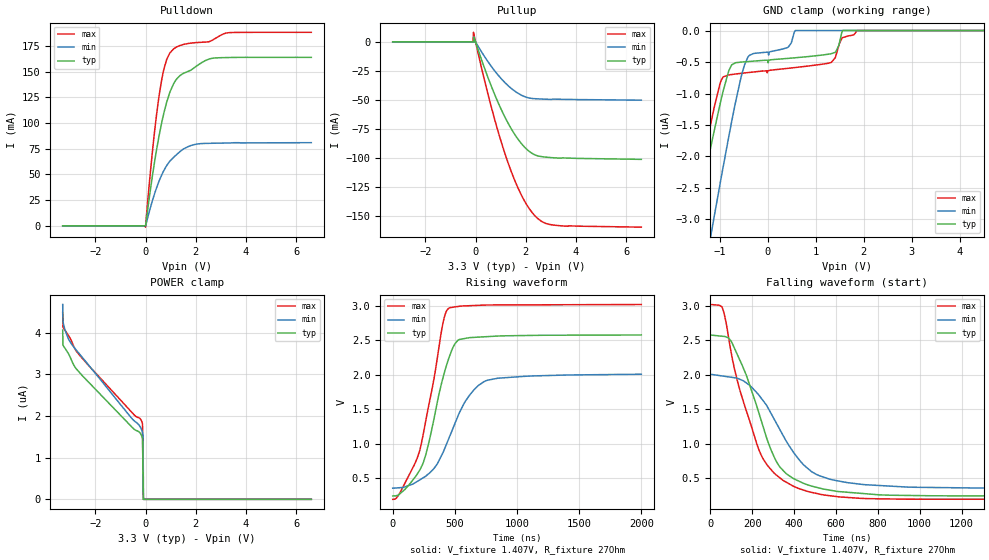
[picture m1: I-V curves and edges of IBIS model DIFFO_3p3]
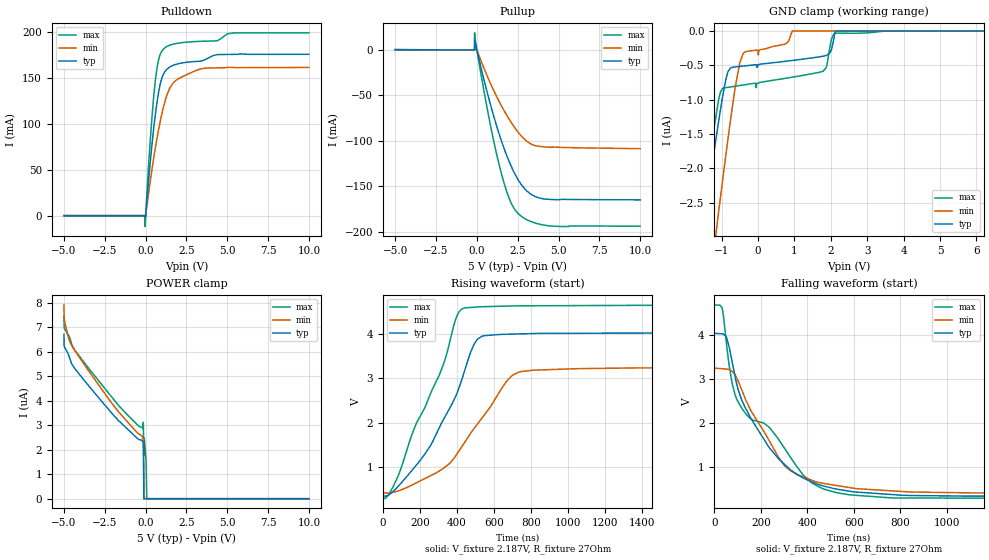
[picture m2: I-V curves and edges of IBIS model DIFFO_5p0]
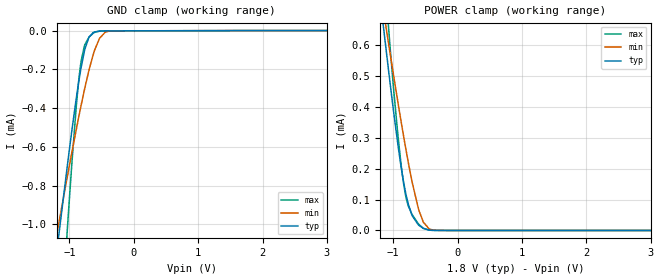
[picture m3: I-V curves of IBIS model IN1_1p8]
|Texas Instruments Incorporated
|ISO1410 5-kVRMS Isolated RS-485/RS-422 Transceiver With Robust EMC
[IBIS Ver]   4.1
[File name]   iso1410.ibs
[Date]   11/07/2018
[File Rev]   1.0
[Source]
| Texas Instruments Incorporated.
| Analog-eLab Design Center, HPA
| 12500 TI Blvd
| Dallas, TX -75243
[Notes]   Revision History:
| Rev 1.0: 11/07/2018
| - Initial version of the model
| - Model generated from simulations in SPECTRE
| - Model names with a trailing _1p8 contain the model for 1.8V operation.
|   Model names with a trailing _2p5 contain the model for 2.5V operation.
|   Model names with a trailing _3p3 contain the model for 3.3V operation.
|   Model names with a trailing _5p0 contain the model for 5.0V operation.
| - C_comp although listed in numerical order of value are
|   obtained from varying PVT conditions. For PVT conditions for
|   each specific value refer the buffer description under
|   respective [Model]. IBIS model user is responsible for using
|   appropriate C_comp to simulate for Signal Integrity.
| - For better transient results, connect a larger capactive load(100n) or
|   connect output common mode node to a constant VCM voltage.
|   typ   min   max
|   PVT 3p3   3.3   3.0   3.6
|   VCM   1.407   1.18047   1.60366
|   PVT 5p0   5.0   4.5   5.5
|   VCM   2.187   1.8289   2.4817
[Disclaimer]
| This model is designed as an aid for customers of Texas Instruments.
| TI and its licensors and suppliers make no warranties, either expressed
| or implied, with respect to this  model, including the warranties of
| merchantability or fitness for a particular purpose. The model is
| provided solely on an "as is" basis. The entire risk as to its quality
| and performance is with the customer.
| This model is subject to change without notice. Texas Instruments
| Incorporated is not responsible for updating this model.
[Copyright]
(C) Copyright 2018 Texas Instruments Incorporated.All rights reserved.
|  Component ISO1410DW 16-Pin SOIC -DW package
|  Part # ISO1410DW
[Component]   ISO1410DW
[Manufacturer]   TI
[Package]   |16 SOIC -DW package
|   typ   min   max
R_pkg   0.05   0.04   0.06
L_pkg   1.0nH   0.8nH   1.2nH
C_pkg   0.2pF   0.16pF   0.24pF
[Pin] signal_name  model_name   R_pin   L_pin   C_pin
1   VCC1   POWER   NA   NA   NA
2   GND1   GND   NA   NA   NA
3   R   OUT   NA   NA   NA
4   REB   IN1   NA   NA   NA
5   DE   IN2   NA   NA   NA
6   D   IN1   NA   NA   NA
7   NC   NC   NA   NA   NA
8   GND1   GND   NA   NA   NA
9   GND2   GND   NA   NA   NA
10   NC   NC   NA   NA   NA
11   NC   NC   NA   NA   NA
12   A   DIFFO   NA   NA   NA
13   B   DIFFO   NA   NA   NA
14   NC   NC   NA   NA   NA
15   GND2   GND   NA   NA   NA
16   VCC2   POWER   NA   NA   NA
[Diff Pin]  inv_pin  vdiff  tdelay_typ tdelay_min tdelay_max
12   13   NA   NA   NA   NA
|  Component ISO1410BDW 16-Pin SOIC -DW package
|  Part # ISO1410BDW
[Component]   ISO1410BDW
[Manufacturer]   TI
[Package]   |16 SOIC -DW package
|   typ   min   max
R_pkg   0.05   0.04   0.06
L_pkg   1.0nH   0.8nH   1.2nH
C_pkg   0.2pF   0.16pF   0.24pF
[Pin] signal_name  model_name   R_pin   L_pin   C_pin
1   VCC1   POWER   NA   NA   NA
2   GND1   GND   NA   NA   NA
3   R   OUT   NA   NA   NA
4   REB   IN1   NA   NA   NA
5   DE   IN2   NA   NA   NA
6   D   IN1   NA   NA   NA
7   NC   NC   NA   NA   NA
8   GND1   GND   NA   NA   NA
9   GND2   GND   NA   NA   NA
10   NC   NC   NA   NA   NA
11   NC   NC   NA   NA   NA
12   A   DIFFO   NA   NA   NA
13   B   DIFFO   NA   NA   NA
14   NC   NC   NA   NA   NA
15   GND2   GND   NA   NA   NA
16   VCC2   POWER   NA   NA   NA
[Diff Pin]  inv_pin  vdiff  tdelay_typ tdelay_min tdelay_max
12   13   NA   NA   NA   NA
|   Model Selectors
[Model Selector] IN1
IN1_1p8   1.8V   digital Input
IN1_2p5   2.5V   digital Input
IN1_3p3   3.3V   digital Input
IN1_5p0   5.0V   digital Input
[Model Selector] IN2
IN2_1p8   1.8V   digital Input
IN2_2p5   2.5V   digital Input
IN2_3p3   3.3V   digital Input
IN2_5p0   5.0V   digital Input
[Model Selector] OUT
OUT_1p8   1.8V   digital Output
OUT_2p5   2.5V   digital Output
OUT_3p3   3.3V   digital Output
OUT_5p0   5.0V   digital Output
[Model Selector] DIFFO
DIFFO_3p3   3.3V   Differential digital Output
DIFFO_5p0   5.0V   Differential digital Output
| Models and submodels in the file (14): DIFFO_3p3 (3-state), DIFFO_5p0 (3-state), IN1_1p8 (Input), IN1_2p5 (Input), IN1_3p3 (Input), IN1_5p0 (Input), IN2_1p8 (Input), IN2_2p5 (Input), IN2_3p3 (Input), IN2_5p0 (Input), OUT_1p8 (3-state), OUT_2p5 (3-state), OUT_3p3 (3-state), OUT_5p0 (3-state)
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|   DIFFO_3p3 Model
[Model]   DIFFO_3p3
Model_type   3-state
Polarity   Non-Inverting
Vmeas = 1.407
Vref = 1.407
Cref = 2pF
Rref = 27
|   typ   min   max
C_comp   26.160pF   24.414pF   26.499pF
|  Where Nom  PVT is Nominal Process, 3.3V,   27C
|   Fast PVT is Strong Process,  3.6,   -40C
|   Slow PVT is Weak Process,   3.0V,   150C
[Voltage Range]   3.3   3   3.6
|Junction temperature
[Temperature Range]   27   150   -40
[Pullup Reference]   3.3   3   3.6
[Pulldown Reference]   0   0   -0
[Power Clamp Reference]   3.3   3   3.6
[GND Clamp Reference]   0   0   0
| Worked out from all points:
|   slope of the pulldown table from 0 to 0.495 V, typ, clamps not added: 6.08 ohm
|   slope of the pullup table from 0 to 0.495 V, typ, clamps not added: 16.1 ohm
|   falling waveform, V_fixture 1.407V, R_fixture 27Ohm: 20-80 % time 166ns typ, 210ns min, 165ns max; typ from 2.58 V to 0.24 V
|   rising waveform, V_fixture 1.407V, R_fixture 27Ohm: 20-80 % time 186ns typ, 258ns min, 187ns max; typ from 0.24 V to 2.58 V
[Pulldown]
|   Voltage   I(typ)   I(min)   I(max)
-3.3V     -2.024nA   -51.84nA   -263.5pA
-3.3mV    291.6nA    408.8nA    -1.354mA
293.7mV   51.97mA    26.12mA    77.15mA
570.9mV   91.69mA    45.41mA    131.6mA
709.5mV   107.6mA    52.85mA    150.1mA
838.2mV   119.9mA    58.43mA    161.5mA
1.125V    138.5mA    66.82mA    172.1mA
1.383V    146.2mA    72.39mA    175.4mA
1.789V    151.1mA    77.87mA    177.6mA
2.65V     162.8mA    80.23mA    180.3mA
3.343V    163.6mA    80.48mA    187.8mA
6.6V      163.8mA    80.8mA     188.1mA
[GND Clamp]
|   Voltage   I(typ)   I(min)   I(max)
-3.3V     -10.21uA   -13.17uA   -10.3uA
-1.627V   -3.473uA   -5.172uA   -3.178uA
-1.251V   -2.072uA   -3.524uA   -1.707uA
-1.142V   -1.677uA   -3.055uA   -1.305uA
-993.3mV  -1.16uA    -2.423uA   -835.8nA
-815.1mV  -640.8nA   -1.688uA   -704.8nA
-419.1mV  -492.9nA   -428.1nA   -668.1nA
570.9mV   -432.4nA   0A         -587.4nA
1.323V    -368nA     0A         -505.4nA
1.561V    0A         0A         -111.9nA
1.858V    0A         0A         0A
6.6V      0A         0A         0A
[Pullup]
|   Voltage   I(typ)   I(min)   I(max)
-3.3V     94.68uA    89.44uA    108uA
-112.2mV  79.61uA    67.94uA    -40.72uA
-102.3mV  79.02uA    67.07uA    89.88uA
-82.5mV   77.83uA    66.27uA    8.407mA
-62.7mV   4.359mA    63.71uA    6.185mA
570.9mV   -34.94mA   -19.25mA   -51.4mA
1.185V    -65.3mA    -35.25mA   -97.06mA
1.68V     -83.38mA   -43.97mA   -125.2mA
2.293V    -96.43mA   -48.67mA   -147.9mA
2.65V     -98.75mA   -49.09mA   -154.8mA
3.066V    -99.61mA   -49.14mA   -157.5mA
6.6V      -101.1mA   -50.04mA   -159.5mA
[POWER Clamp]
|   Voltage   I(typ)   I(min)   I(max)
-3.3V     4.061uA    4.674uA    4.484uA
-3.29V    3.704uA    4.279uA    4.135uA
-3.27V    3.681uA    4.211uA    4.113uA
-3.003V   3.411uA    3.774uA    3.863uA
-2.845V   3.206uA    3.644uA    3.648uA
-2.597V   3.02uA     3.463uA    3.435uA
-161.7mV  1.531uA    1.673uA    1.882uA
-122.1mV  1.452uA    1.601uA    1.799uA
-102.3mV  711.8nA    1.552uA    308.9nA
-92.4mV   0A         776nA      154.5nA
-82.5mV   0A         0A         0A
6.6V      0A         0A         0A
[Ramp]
R_load = 27
|   typ   min   max
dV/dt_r   1.40083/1.85735e-07   0.991895/2.57165e-07   1.69534/1.86502e-07
dV/dt_f   1.40085/1.65885e-07   0.991916/2.08425e-07   1.69537/1.64659e-07
[Falling Waveform]
V_fixture = 1.407V
V_fixture_min = 1.18V
V_fixture_max = 1.604V
R_fixture = 27Ohm
C_fixture = 0F
|   Time   V(typ)   V(min)   V(max)
0s        2.575V     2.006V     3.017V
59.81ns   2.556V     1.98V      2.952V
97.3ns    2.495V     1.963V     2.362V
130.4ns   2.283V     1.946V     1.897V
242.3ns   1.345V     1.663V     838.7mV
317.9ns   728.9mV    1.284V     538.7mV
396.6ns   493.8mV    877.7mV    382.4mV
519ns     356.8mV    536.7mV    269mV
734.9ns   274.6mV    404.8mV    204.1mV
2us       240.5mV    352.8mV    191.8mV
[Rising Waveform]
V_fixture = 1.407V
V_fixture_min = 1.18V
V_fixture_max = 1.604V
R_fixture = 27Ohm
C_fixture = 0F
|   Time   V(typ)   V(min)   V(max)
0s        240.4mV    352.8mV    191.8mV
60.7ns    277mV      360.9mV    294.7mV
214.2ns   606.6mV    470.1mV    879.8mV
265.9ns   836.5mV    528.5mV    1.33V
406.3ns   1.967V     877.2mV    2.765V
447.2ns   2.217V     1.056V     2.958V
531.2ns   2.506V     1.427V     2.99V
653ns     2.541V     1.778V     3.002V
764.3ns   2.552V     1.92V      3.01V
2us       2.575V     2.006V     3.017V
|   DIFFO_5p0 Model
[Model]   DIFFO_5p0
Model_type   3-state
Polarity   Non-Inverting
Vmeas = 2.187
Vref = 2.187
Cref = 2pF
Rref = 27
|   typ   min   max
C_comp   23.969pF   22.997pF   24.641pF
|  Where Nom  PVT is Nominal Process, 5.0V,   27C
|   Fast PVT is Strong Process,  5.5,   -40C
|   Slow PVT is Weak Process,   4.5V,   150C
[Voltage Range]   5   4.5   5.5
|Junction Temperature
[Temperature Range]   27   150   -40
[Pullup Reference]   5   4.5   5.5
[Pulldown Reference]   0   0   0
[Power Clamp Reference]   5   4.5   5.5
[GND Clamp Reference]   0   0   0
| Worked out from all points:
|   slope of the pulldown table from 0 to 0.75 V, typ, clamps not added: 5.76 ohm
|   slope of the pullup table from 0 to 0.75 V, typ, clamps not added: 13.7 ohm
|   falling waveform, V_fixture 2.187V, R_fixture 27Ohm: 20-80 % time 219ns typ, 190ns min, 283ns max; typ from 4.04 V to 0.339 V
|   rising waveform, V_fixture 2.187V, R_fixture 27Ohm: 20-80 % time 263ns typ, 299ns min, 246ns max; typ from 0.339 V to 4.04 V
[Pulldown]
|   Voltage   I(typ)   I(min)   I(max)
-5V       -2.768nA   -62.41nA   -404.6pA
-50mV     415.5nA    532.5nA    -31.17uA
-35mV     425.9nA    562.9nA    -11.95mA
-5mV      -1.626mA   644.3nA    -2.237mA
280mV     57.58mA    36.83mA    80.9mA
610mV     112.3mA    75.29mA    149.5mA
865mV     141.1mA    100.3mA    174.6mA
1.21V     157.9mA    126.3mA    183.7mA
1.78V     164.7mA    146.5mA    187.6mA
3.34V     168.6mA    160mA      190.3mA
5.38V     176.1mA    161.9mA    199.5mA
10V       176.2mA    161.8mA    199.6mA
[GND Clamp]
|   Voltage   I(typ)   I(min)   I(max)
-5V       -16.78uA   -20.83uA   -17.26uA
-1.595V   -3.188uA   -4.867uA   -2.896uA
-1.235V   -1.86uA    -3.297uA   -1.512uA
-1.04V    -1.18uA    -2.463uA   -908.9nA
-830mV    -603.4nA   -1.596uA   -820.5nA
-620mV    -522.8nA   -806.6nA   -803.4nA
-410mV    -510.7nA   -331.6nA   -786.3nA
940mV     -428.8nA   0A         -672.2nA
1.795V    -366.7nA   0A         -583.8nA
1.99V     -304.5nA   0A         -189.9nA
2.14V     0A         0A         -30.64nA
10V       0A         0A         0A
[Pullup]
|   Voltage   I(typ)   I(min)   I(max)
-5V       407.4uA    275.7uA    569.2uA
-155mV    86.47uA    72.78uA    97.97uA
-140mV    85.13uA    71.46uA    19mA
-110mV    10.37mA    70.25uA    12.13mA
-80mV     6.404mA    4.087mA    8.829mA
730mV     -53.4mA    -32.7mA    -73.69mA
1.45V     -97.33mA   -59.72mA   -132.6mA
2.08V     -127.2mA   -79.16mA   -167.8mA
2.725V    -148.3mA   -94.82mA   -183.3mA
3.34V     -159.2mA   -103.8mA   -189.2mA
4.18V     -164.2mA   -106.7mA   -193.1mA
10V       -165.1mA   -108.7mA   -194.1mA
[POWER Clamp]
|   Voltage   I(typ)   I(min)   I(max)
-5V       6.707uA    7.907uA    7.452uA
-4.94V    6.153uA    7.179uA    6.91uA
-4.49V    5.463uA    6.208uA    6.246uA
-170mV    2.317uA    2.48uA     2.877uA
-140mV    2.26uA     2.422uA    3.117uA
-125mV    1.13uA     2.386uA    2.344uA
-110mV    0A         1.193uA    1.76uA
-95mV     0A         0A         2.476uA
25mV      0A         0A         1.572uA
70mV      0A         0A         32.08nA
100mV     0A         0A         0A
10V       0A         0A         0A
[Ramp]
R_load = 27
|   typ   min   max
dV/dt_r   2.21767/2.62862e-07   1.70352/2.97953e-07   2.6284/2.46502e-07
dV/dt_f   2.2197/2.17013e-07   1.70411/1.8988e-07   2.64089/2.82769e-07
[Falling Waveform]
V_fixture = 2.187V
V_fixture_min = 1.829V
V_fixture_max = 2.482V
R_fixture = 27Ohm
C_fixture = 0F
|   Time   V(typ)   V(min)   V(max)
0s        4.038V     3.249V     4.684V
33.14ns   4.028V     3.235V     4.624V
51.97ns   3.952V     3.226V     3.833V
74.4ns    3.456V     3.186V     2.972V
109.7ns   2.649V     2.864V     2.411V
231.5ns   1.481V     1.644V     1.926V
299.4ns   1.076V     1.052V     1.449V
457.8ns   588.2mV    640.7mV    530.4mV
764.5ns   376.4mV    459.9mV    299.4mV
2us       338.6mV    409.1mV    282.3mV
[Rising Waveform]
V_fixture = 2.187V
V_fixture_min = 1.829V
V_fixture_max = 2.482V
R_fixture = 27Ohm
C_fixture = 0F
|   Time   V(typ)   V(min)   V(max)
0s        338.6mV    409mV      282.3mV
81.44ns   558.1mV    457.4mV    792mV
254.5ns   1.466V     797.2mV    2.63V
330.8ns   2.101V     981.7mV    3.368V
395.8ns   2.621V     1.266V     4.37V
430.6ns   3.032V     1.487V     4.58V
511.9ns   3.89V      1.976V     4.617V
673.1ns   4V         2.959V     4.637V
738.7ns   4.007V     3.147V     4.643V
2us       4.035V     3.248V     4.663V
|   IN1_1p8 Model
[Model]   IN1_1p8
Model_type   Input
Vinl = 0.54
Vinh = 1.26
|   typ   min   max
C_comp   0.00095pF   0.00076pF   0.0142pF
|  Where Nom  PVT is Nominal Process, 1.8V,  27C
|   Fast PVT is Strong Process,  1.89,  -40C
|   Slow PVT is Weak Process,   1.71V, 150C
[Model spec]
|subparameter
Vinl   0.54   0.513   0.567
Vinh   1.26   1.197   1.323
[Voltage Range]   1.8   1.71   1.89
|Junction Temperature
[Temperature Range]   27   150   -40
[Power Clamp Reference]   1.8   1.71   1.89
[GND Clamp Reference]   0   0   0
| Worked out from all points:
|   GND clamp passes 1 mA (typ) near -1.14 V on its own axis
|   POWER clamp passes 1 mA (typ) near -1.34 V on its own axis
[GND Clamp]
|   Voltage   I(typ)   I(min)   I(max)
-1.8V     -2.874mA   -2.195mA   -5.336mA
-1.184V   -1.11mA    -1.03mA    -1.821mA
-1.163V   -1.051mA   -990.6uA   -1.705mA
-1.028V   -686uA     -745.6uA   -1.004mA
-898.2mV  -361.3uA   -518.9uA   -411.1uA
-828mV    -209.5uA   -402uA     -181.4uA
-757.8mV  -93.79uA   -292.1uA   -71.12uA
-698.4mV  -36.2uA    -207.5uA   -35.59uA
-633.6mV  -10.97uA   -127.9uA   -14.52uA
-531mV    -2.469uA   -39.62uA   -2.975uA
-369mV    -1.445uA   -2.669uA   -1.543uA
3.6V      0A         0A         0A
[POWER Clamp]
|   Voltage   I(typ)   I(min)   I(max)
-1.8V     1.872mA    1.618mA    2.869mA
-1.179V   709.8uA    751.5uA    957.6uA
-1.055V   490uA      584.3uA    612.9uA
-919.8mV  269uA      408.1uA    296.9uA
-871.2mV  199.5uA    346.9uA    204.2uA
-817.2mV  133.9uA    281.2uA    125.6uA
-768.6mV  88.65uA    224.9uA    81.75uA
-703.8mV  48uA       155.6uA    51.14uA
-612mV    19.26uA    74.45uA    22.69uA
-531mV    6.785uA    27.03uA    7.136uA
-293.4mV  209.8nA    425.9nA    202.8nA
3.6V      0A         0A         0A
